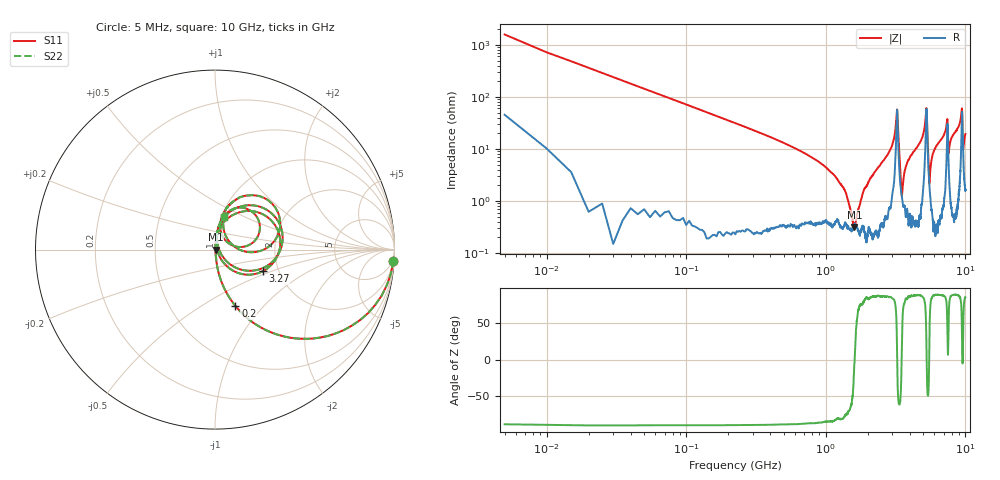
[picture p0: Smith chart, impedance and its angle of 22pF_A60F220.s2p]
! Amotech Co.,Ltd.
! http://www.amotech.co.kr/
! Part Number: A60F220
! These Parameters are Measured in Series Mode Connection
! Operation Temp=25[degC], DC Bias Voltage=0[V]
! Freq. Start=5[MHz] Stop=10[GHz], 2000[Steps]
! Date: Monday, July 20, 2020, 03:37:15
# GHZ S RI R 50.000000
!Freq.(Hz) S11(Real) S11(Imag) S21(Real) S21(Imag) S12(Real) S12(Imag) S22(Real) S22(Imag)
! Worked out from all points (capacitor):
!   2000 points, 5 MHz to 10 GHz, reference 50 ohm
!   read as one part in series: C = 22.1 pF near 55 MHz
!   lowest |Z| = 318 mohm at 1.605 GHz (marker M1)
!   series resonance near 1.609 GHz, so ESL is about 440 pH
!   S11 on the Smith chart (normalised r, x): 5 MHz: 2, -32; 200 MHz: 1.00, -0.71; 3.27 GHz: 1.65, -0.44; 10 GHz: 1.03, +0.39
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0.005  0.9942 -0.0626  0.00575 0.0626  0.00575 0.0626  0.9942 -0.0626
0.075  0.4781 -0.4962  0.5219 0.4962  0.5219 0.4962  0.4781 -0.4962
0.2  0.1141 -0.3146  0.8859 0.3146  0.8859 0.3146  0.1141 -0.3146
1.325  0.00328 -0.0182  0.9967 0.0182  0.9967 0.0182  0.00328 -0.0182
1.605  0.00316 -0.000282  0.9968 0.000282  0.9968 0.000282  0.00316 -0.000282
1.675  0.00317 0.00467  0.9968 -0.00467  0.9968 -0.00467  0.00317 0.00467
2.055  0.00358 0.0253  0.9964 -0.0253  0.9964 -0.0253  0.00358 0.0253
3.27  0.2659 -0.1212  0.7341 0.1212  0.7341 0.1212  0.2659 -0.1212
3.34  0.0634 -0.0894  0.9366 0.0894  0.9366 0.0894  0.0634 -0.0894
3.51  0.0117 0.00475  0.9883 -0.00475  0.9883 -0.00475  0.0117 0.00475
3.85  0.00931 0.0556  0.9907 -0.0556  0.9907 -0.0556  0.00931 0.0556
5.005  0.0547 0.1829  0.9453 -0.1829  0.9453 -0.1829  0.0547 0.1829
5.27  0.3712 0.0194  0.6288 -0.0194  0.6288 -0.0194  0.3712 0.0194
5.525  0.0188 0.00973  0.9812 -0.00973  0.9812 -0.00973  0.0188 0.00973
5.835  0.0105 0.078  0.9895 -0.078  0.9895 -0.078  0.0105 0.078
6.67  0.027 0.1455  0.973 -0.1455  0.973 -0.1455  0.027 0.1455
7.4  0.2145 0.2043  0.7855 -0.2043  0.7855 -0.2043  0.2145 0.2043
7.585  0.0511 0.0593  0.9489 -0.0593  0.9489 -0.0593  0.0511 0.0593
8.335  0.044 0.1936  0.956 -0.1936  0.956 -0.1936  0.044 0.1936
9.405  0.3198 0.2542  0.6802 -0.2542  0.6802 -0.2542  0.3198 0.2542
9.64  0.0753 0.0504  0.9247 -0.0504  0.9247 -0.0504  0.0753 0.0504
10  0.0504 0.1801  0.9496 -0.1801  0.9496 -0.1801  0.0504 0.1801
